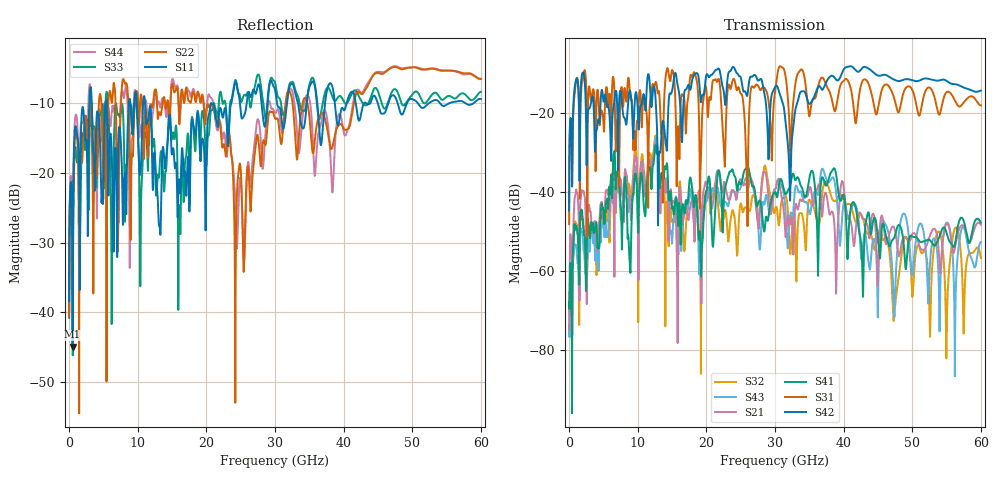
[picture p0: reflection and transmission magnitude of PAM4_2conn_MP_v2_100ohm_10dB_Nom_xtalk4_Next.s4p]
! Info: Touchstone file created by Circ.  Input file=FAB50GbE_2conn_Midplane_Examax_Topo2_v2_100ohm_10dB_Nom.circ
# Hz S RI R 50
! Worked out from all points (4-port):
!   6000 points, 10 MHz to 60 GHz, reference 50 ohm
!   strongest paths, dB at 10 MHz, 15.01 GHz, 30.01 GHz, 45.01 GHz, 60 GHz:
!     S42: -44.6, -14.5, -13.5, -10.6, -14.4
!     S31: -48.1, -9.2, -14.8, -18.9, -18.1
!     S41: -67.8, -44.0, -40.0, -51.4, -47.8
!     S21: -74.8, -42.9, -39.4, -61.1, -48.3
!     S43: -70.8, -53.0, -39.2, -68.7, -52.7
!     S32: -74.3, -47.3, -44.9, -50.9, -56.7
!   lowest |S11| = -44.9 dB at 520 MHz (marker M1), VSWR 1.01, Z = 49.4 + j0.0383 ohm
!   |S11| at or under -10 dB: start of sweep to 2.959 GHz; 5.437 GHz to 8.718 GHz (3.282 GHz wide, 46.4 % of centre); 11.07 GHz to 23.64 GHz (12.57 GHz wide, 72.4 % of centre)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
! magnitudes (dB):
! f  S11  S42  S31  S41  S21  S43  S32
! 10 MHz  -38.4  -44.6  -48.1  -67.8  -74.8  -70.8  -74.3
! 520 MHz  -44.9  -24.7  -27.1  -57.1  -56.9  -62.8  -60.6
! 12.64 GHz  -20.3  -17.6  -12.2  -28.3  -28.2  -26.4  -25.9
! 19.18 GHz  -18.1  -17.2  -32.8  -56.6  -47.0  -50.4  -68.1
! 28.56 GHz  -13.3  -16.0  -13.9  -48.4  -35.0  -42.2  -33.4
! 47.38 GHz  -8.9  -11.7  -16.4  -51.5  -49.1  -71.5  -71.3
! 60 GHz  -9.4  -14.4  -18.1  -47.8  -48.3  -52.7  -56.7
